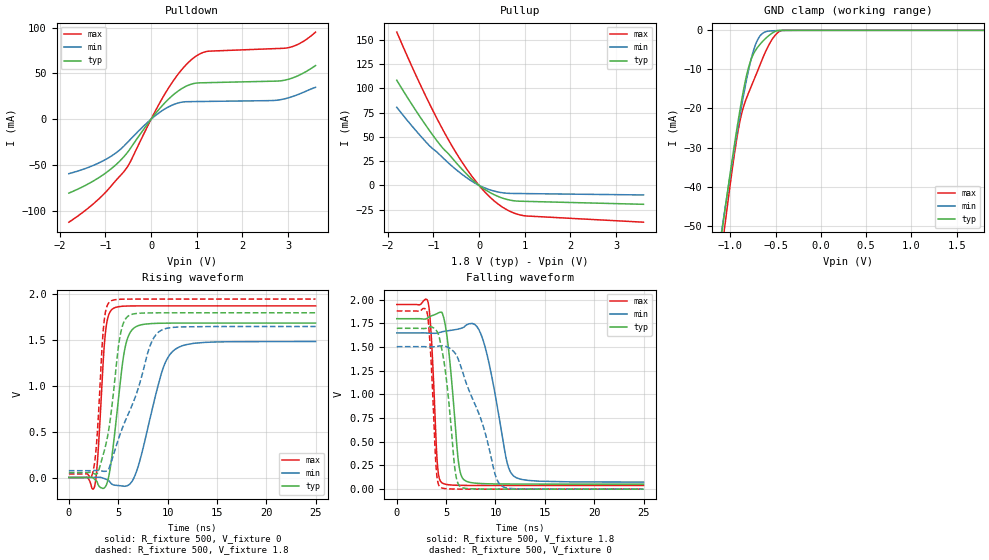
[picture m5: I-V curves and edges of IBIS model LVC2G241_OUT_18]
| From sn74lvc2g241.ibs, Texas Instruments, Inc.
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[Model]   LVC2G241_OUT_18
Model_type  3-state
Enable   Active-High
Vref =   0
Rref =   1k
Cref =   30p
Vmeas =   0.9
| variable   typ   min   max
C_comp   6.12pF   5.33pF   6.95pF
| C_pullup   9.53pF   6.44pF   11.63pF
| C_pulldown   10.66pF   6.75pF   16.56pF
| C_tri-state   6.12pF   5.33pF   6.95pF
[Temperature Range]   40   100   -40
| Ambient temperature   25   85   -40
[Voltage range]   1.8   1.65   1.95
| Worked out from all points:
|   slope of the pulldown table from 0 to 0.27 V, typ, clamps not added: 16.6 ohm
|   slope of the pullup table from 0 to 0.27 V, typ, clamps not added: 33.1 ohm
|   GND clamp passes 1 mA (typ) near -0.56 V on its own axis
|   rising waveform, R_fixture 500, V_fixture 0: 20-80 % time 1.09ns typ, 2.07ns min, 612ps max; typ from 0 V to 1.69 V
|   falling waveform, R_fixture 500, V_fixture 1.8: 20-80 % time 861ps typ, 1.63ns min, 501ps max; typ from 1.8 V to 0.054 V
|   rising waveform, R_fixture 500, V_fixture 1.8: 20-80 % time 1.21ns typ, 2.99ns min, 614ps max; typ from 0.054 V to 1.8 V
|   falling waveform, R_fixture 500, V_fixture 0: 20-80 % time 993ps typ, 2.86ns min, 513ps max; typ from 1.7 V to 0 V
[GND Clamp]
| LVC2G241_OUT_18
|   Voltage   I(typ)   I(min)   I(max)
-1.8V     -180mA     -169.8mA   -199.3mA
-1.09V    -50.88mA   -50.27mA   -55.25mA
-1.055V   -45.05mA   -44.88mA   -48.78mA
-920mV    -23.93mA   -25.13mA   -26.38mA
-875mV    -17.74mA   -19.11mA   -21.2mA
-820mV    -11.37mA   -12.4mA    -17.19mA
-775mV    -7.672mA   -7.713mA   -14.61mA
-725mV    -5.204mA   -3.777mA   -11.81mA
-630mV    -2.493mA   -554uA     -6.414mA
-530mV    -582.7uA   -113.1uA   -1.993mA
-430mV    -5.996uA   -38.12uA   -30.78uA
1.8V      20.22pA    26.25nA    581.3pA
[Pulldown]
| LVC2G241_OUT_18
|   Voltage   I(typ)   I(min)   I(max)
-1.8V     -80.79mA   -59.53mA   -112.6mA
-1.085V   -61.95mA   -46.38mA   -84.36mA
-570mV    -39.5mA    -28.12mA   -55.7mA
-445mV    -31.3mA    -21.63mA   -45.66mA
-35mV     -2.334mA   -1.547mA   -3.49mA
330mV     19.4mA     12.06mA    29.99mA
640mV     32.46mA    18.32mA    52.36mA
930mV     39mA       19.26mA    67.03mA
1.25V     39.98mA    19.47mA    74.33mA
2.865V    42.16mA    21.66mA    77.49mA
3.215V    47.55mA    26.98mA    81.88mA
3.6V      58.7mA     34.88mA    95.26mA
[Pullup]
| LVC2G241_OUT_18
|   Voltage   I(typ)   I(min)   I(max)
-1.8V     108.2mA    80.38mA    157.8mA
-1.425V   80.1mA     58.76mA    117.9mA
-1.08V    56.19mA    40.61mA    83.64mA
-815mV    39.58mA    29.51mA    59.35mA
-595mV    28.49mA    19.95mA    40.88mA
-320mV    14.01mA    9.554mA    20.26mA
-45mV     1.662mA    1.097mA    2.622mA
175mV     -5.605mA   -3.539mA   -9.138mA
400mV     -11.07mA   -6.643mA   -18.6mA
700mV     -15.37mA   -8.29mA    -27.23mA
1V        -16.44mA   -8.458mA   -31.32mA
3.6V      -19.49mA   -9.866mA   -37.91mA
[Ramp]
| LVC2G241_OUT_18
| variable   typ   min   max
dV/dt_r   1.08/1.17E-09   0.95/2.19E-09   1.20/6.56E-10
dV/dt_f   1.09/9.11E-10   1.01/1.77E-09   1.18/5.26E-10
R_load = 500
[Rising Waveform]
| LVC2G241_OUT_18
R_fixture =   500
C_fixture =   0
L_fixture =   0
V_fixture =   0
V_fixture_min = 0
V_fixture_max = 0
|   Time   V(typ)   V(min)   V(max)
0s        111.1pV    7.577nV    2.783nV
2.605ns   -18.45mV   2.041mV    -98.12mV
2.93ns    -67.64mV   3.202mV    227.3mV
3.69ns    -102.2mV   -15.42mV   1.566V
4.46ns    313.2mV    -78.7mV    1.845V
5.625ns   1.38V      -95.92mV   1.873V
6.72ns    1.643V     27.65mV    1.875V
9.45ns    1.686V     1.163V     1.876V
10.74ns   1.687V     1.398V     1.876V
24.99ns   1.688V     1.486V     1.876V
[Falling Waveform]
| LVC2G241_OUT_18
R_fixture =   500
C_fixture =   0
L_fixture =   0
V_fixture =   1.8
V_fixture_min = 1.65
V_fixture_max = 1.95
|   Time   V(typ)   V(min)   V(max)
0s        1.8V       1.65V      1.95V
3.165ns   1.81V      1.648V     1.977V
4.105ns   1.856V     1.648V     277.4mV
4.575ns   1.866V     1.661V     66.96mV
5.25ns    1.473V     1.674V     46.54mV
6.265ns   276.3mV    1.692V     40.61mV
6.82ns    97.43mV    1.712V     39.72mV
8.71ns    58.67mV    1.584V     38.94mV
11.83ns   54.11mV    139.6mV    38.84mV
24.99ns   53.62mV    74.79mV    38.83mV
[Rising Waveform]
| LVC2G241_OUT_18
R_fixture =   500
C_fixture =   0
L_fixture =   0
V_fixture =   1.8
V_fixture_min = 1.65
V_fixture_max = 1.95
|   Time   V(typ)   V(min)   V(max)
0s        53.59mV    74.64mV    38.81mV
2.45ns    49.19mV    75.29mV    67.9mV
2.835ns   39.85mV    77.19mV    414.2mV
3.535ns   271.2mV    67.4mV     1.668V
4.19ns    632.1mV    139mV      1.925V
5.04ns    1.445V     425.3mV    1.947V
5.6ns     1.706V     589.2mV    1.949V
8.25ns    1.799V     1.445V     1.95V
9.225ns   1.8V       1.6V       1.95V
24.99ns   1.8V       1.65V      1.95V
[Falling Waveform]
| LVC2G241_OUT_18
R_fixture =   500
C_fixture =   0
L_fixture =   0
V_fixture =   0
V_fixture_min = 0
V_fixture_max = 0
|   Time   V(typ)   V(min)   V(max)
0s        1.699V     1.505V     1.882V
3.055ns   1.703V     1.503V     1.871V
3.43ns    1.714V     1.503V     1.436V
3.99ns    1.677V     1.506V     222.9mV
4.41ns    1.553V     1.514V     20.07mV
5.06ns    1.131V     1.504V     4.437mV
5.915ns   192.5mV    1.435V     1.005mV
6.44ns    26.55mV    1.31V      479.3uV
10.64ns   227.5uV    32.39mV    26.62uV
24.99ns   23.52uV    48.06uV    15.81uV
